(* Logix 5000 AddOnInstructionDefinition export AMCI_SV160E2_Home_CCW; software revision 20.03 *)

ADD_ON_INSTRUCTION AMCI_SV160E2_Home_CCW   (* revision 1.0, vendor AMCI, ExecuteEnableInFalse *)
// Revision note:
// 8/2019 Version 0 Initial release of SV160E2 Add On Instructions.
// 3/17/20 Version 1 replaced the generic EDS file with a more complete V1.6 EDS file.
VAR_INPUT
   Status_Word_0 : INT; {required}
        .0   // Set when the SV160E2 is moving CW
        .1   // Set when SV160E2 is moving CCW
        .7   // SV160E2 Move Complete bit
        .11   // Set when there is an input error
        .12   // set when there is a command error
        .13   // set when there is a configuration error
   Status_Word_1 : INT; {required}
        .15   // Set when SV160E2 is enabled
   Programmed_Speed : DINT; {required}
   Acceleration : INT; {required}
   Deceleration : INT; {required}
   Maximum_Move_Torque : INT;
END_VAR
VAR_IN_OUT
   AMCI_SV160E2_output_data : _000A:SV160E2_9125ACD4:O:0; {required}
END_VAR
VAR_OUTPUT
   EN : BOOL; {access Read Only, visible}   // AOI EN bit
   ER : BOOL; {access Read Only, visible}   // AOI ER bit
END_VAR
VAR
   command_data_block : INT[10];
        [0]   // Command Word 0
        [1]   // Command Word 1
        [2]   // Upper Target Position
        [3]   // Lower Target Position
        [4]   // Upper Programmed Speed
        [5]   // Lower Programmed Speed
END_VAR

ROUTINE EnableInFalse   (* ladder *)
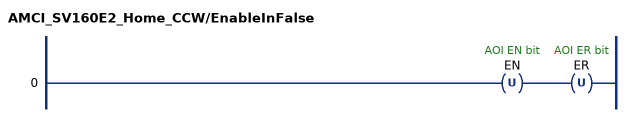
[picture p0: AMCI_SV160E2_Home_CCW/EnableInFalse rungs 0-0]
   0: OTU(EN)OTU(ER);
END_ROUTINE

ROUTINE Logic   (* ladder *)
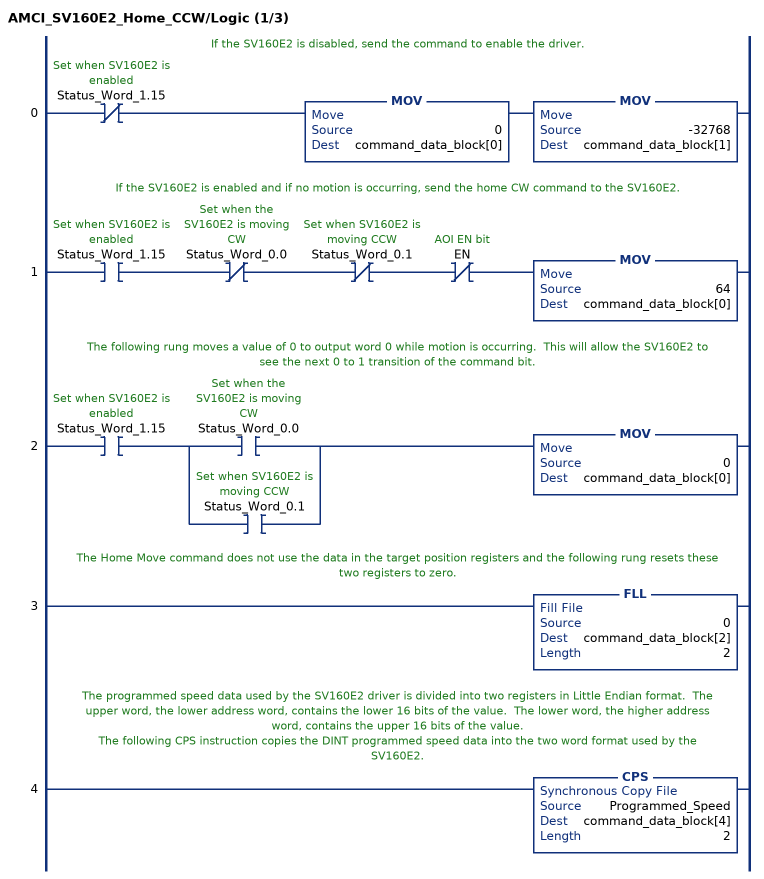
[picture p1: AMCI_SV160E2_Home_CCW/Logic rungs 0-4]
   // If the SV160E2 is disabled, send the command to enable the driver.
   0: XIO(Status_Word_1.15)MOV(0,command_data_block[0])MOV(-32768,command_data_block[1]);
   // If the SV160E2 is enabled and if no motion is occurring, send the home CW command to the SV160E2.
   1: XIC(Status_Word_1.15)XIO(Status_Word_0.0)XIO(Status_Word_0.1)XIO(EN)MOV(64,command_data_block[0]);
   // The following rung moves a value of 0 to output word 0 while motion is occurring.  This will allow the SV160E2 to see the next 0 to 1 transition of the command bit.
   2: XIC(Status_Word_1.15)[XIC(Status_Word_0.0) ,XIC(Status_Word_0.1) ]MOV(0,command_data_block[0]);
   // The Home Move command does not use the data in the target position registers and the following rung resets these two registers to zero.
   3: FLL(0,command_data_block[2],2);
   // The programmed speed data used by the SV160E2 driver is divided into two registers in Little Endian format.  The upper word, the lower address word, contains the lower 16 bits of the value.  The lower word, the higher address word, contains the upper 16 bits of the value.
   // The following CPS instruction copies the DINT programmed speed data into the two word format used by the SV160E2.
   4: CPS(Programmed_Speed,command_data_block[4],2);
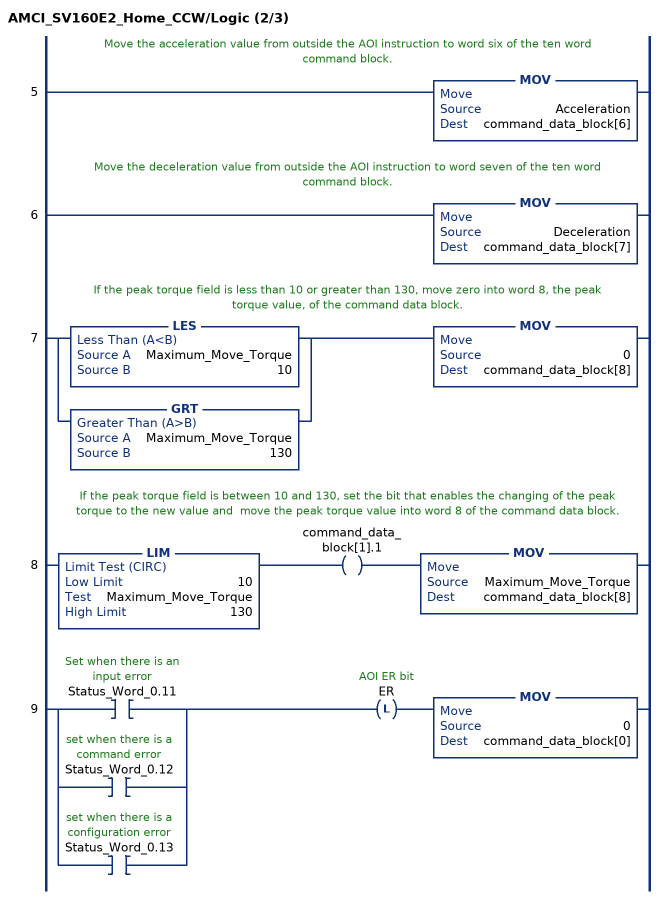
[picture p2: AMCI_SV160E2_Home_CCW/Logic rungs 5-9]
   // Move the acceleration value from outside the AOI instruction to word six of the ten word command block.
   5: MOV(Acceleration,command_data_block[6]);
   // Move the deceleration value from outside the AOI instruction to word seven of the ten word command block.
   6: MOV(Deceleration,command_data_block[7]);
   // If the peak torque field is less than 10 or greater than 130, move zero into word 8, the peak torque value, of the command data block.
   7: [LES(Maximum_Move_Torque,10) ,GRT(Maximum_Move_Torque,130) ]MOV(0,command_data_block[8]);
   // If the peak torque field is between 10 and 130, set the bit that enables the changing of the peak torque to the new value and  move the peak torque value into word 8 of the command data block.
   8: LIM(10,Maximum_Move_Torque,130)OTE(command_data_block[1].1)MOV(Maximum_Move_Torque,command_data_block[8]);
   9: [XIC(Status_Word_0.11) ,XIC(Status_Word_0.12) ,XIC(Status_Word_0.13) ]OTL(ER)MOV(0,command_data_block[0]);
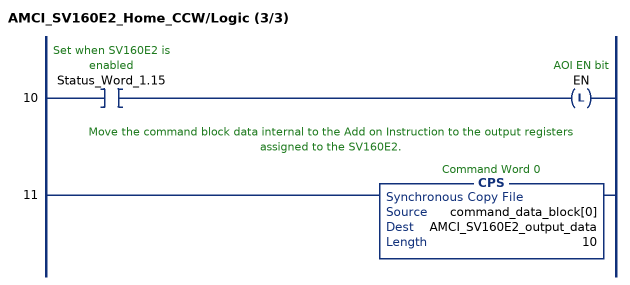
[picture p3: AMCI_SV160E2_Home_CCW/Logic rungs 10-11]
   10: XIC(Status_Word_1.15)OTL(EN);
   // Move the command block data internal to the Add on Instruction to the output registers assigned to the SV160E2.
   11: CPS(command_data_block[0],AMCI_SV160E2_output_data,10);
END_ROUTINE
END_ADD_ON_INSTRUCTION
